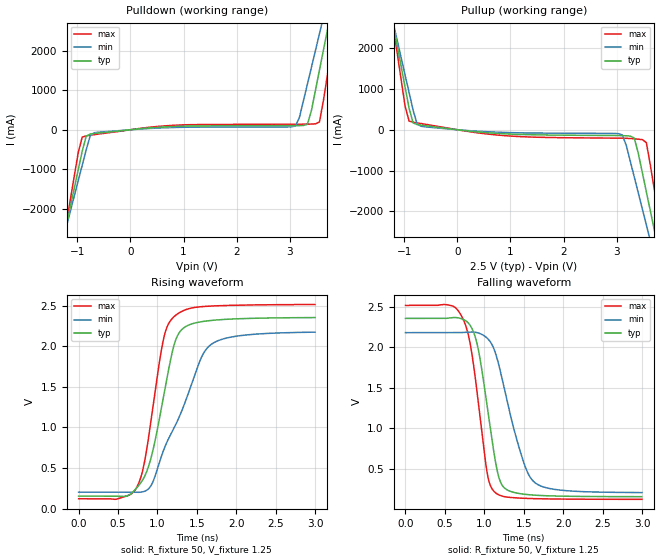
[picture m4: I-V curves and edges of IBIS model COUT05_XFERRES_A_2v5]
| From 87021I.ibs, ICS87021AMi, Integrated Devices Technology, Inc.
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[Model] COUT05_XFERRES_A_2v5
Model_type  Output
Polarity   Non-Inverting
Vmeas = 1.25
Rref = 50
Cref = 0
Vref = 1.25
|Variable  typ   min   max
C_comp   2p   1.5p   2.5p
[Voltage Range]   2.5   2.375   2.625
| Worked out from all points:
|   slope of the pulldown table from 0 to 0.375 V, typ, clamps not added: 7.84 ohm
|   slope of the pullup table from 0 to 0.375 V, typ, clamps not added: 7.17 ohm
|   rising waveform, R_fixture 50, V_fixture 1.25: 20-80 % time 274ps typ, 488ps min, 225ps max; typ from 0.154 V to 2.35 V
|   falling waveform, R_fixture 50, V_fixture 1.25: 20-80 % time 205ps typ, 309ps min, 191ps max; typ from 2.35 V to 0.154 V
| Open source, no load
|  Voltage   I(typ)   I(min)   I(max)
[Pullup]
-2.5V     11.44A     9.986A     13.84A
-1.212V   2.607A     2.64A      2.573A
-909.1mV  526mA      911.1mA    212mA
-833.3mV  167.1mA    478.9mA    184.4mA
-681.8mV  112.7mA    84.76mA    151.8mA
3.106V    -144.5mA   -124.8mA   -207.2mA
3.333V    -201.9mA   -1.16A     -222.3mA
3.485V    -1.051A    -1.943A    -242.2mA
3.561V    -1.521A    -2.334A    -315mA
3.712V    -2.464A    -3.118A    -1.472A
3.864V    -3.407A    -3.903A    -2.677A
5V        -10.49A    -9.798A    -11.71A
[Pulldown]
-2.5V     -10.49A    -9.183A    -12.66A
-1.288V   -2.917A    -2.872A    -3.01A
-1.212V   -2.443A    -2.477A    -2.405A
-909.1mV  -543.8mA   -898.7mA   -186.9mA
-833.3mV  -160.7mA   -504.4mA   -155.1mA
-757.6mV  -109mA     -149.4mA   -139.6mA
3.106V    103.9mA    93.06mA    139.6mA
3.333V    137.9mA    1.155A     141.5mA
3.561V    1.512A     2.434A     197.9mA
3.712V    2.539A     3.288A     1.405A
3.864V    3.567A     4.143A     2.72A
5V        11.31A     10.58A     12.63A
[Ramp]
|   typ   min   max
dV/dt_r   1.762/0.433n   1.577/0.660n   1.919/0.360n
dV/dt_f   1.769/0.311n   1.585/0.457n   1.923/0.297n
R_load =   50.0000
[Rising Waveform]
R_fixture = 50
V_fixture = 1.25   | VCC_typ
V_fixture_max = 1.3125   | VCC_max
V_fixture_min = 1.1875   | VCC_min
C_fixture = 0.0p
| Time   typ   min   max
0s        154.1mV    203.2mV    121.3mV
477.4ps   154.3mV    203.2mV    116.6mV
740.9ps   259.7mV    200.8mV    269.6mV
821.5ps   368.8mV    208.9mV    507.2mV
905.2ps   578.3mV    264.4mV    996.6mV
1.079ns   1.39V      722.9mV    2.098V
1.228ns   2.067V     1.027V     2.379V
1.553ns   2.301V     1.854V     2.487V
1.693ns   2.318V     2.03V      2.495V
2.998ns   2.352V     2.173V     2.513V
[Falling Waveform]
R_fixture = 50
V_fixture = 1.25   | VCC_typ
V_fixture_max = 1.3125   | VCC_max
V_fixture_min = 1.1875   | VCC_min
C_fixture = 0.0p
| Time   typ   min   max
0s        2.355V     2.179V     2.515V
725.4ps   2.344V     2.181V     2.356V
818.4ps   2.271V     2.187V     2.053V
911.4ps   2.026V     2.178V     1.415V
1.039ns   1.249V     2.109V     432mV
1.141ns   587mV      1.926V     202.8mV
1.259ns   258.4mV    1.464V     154.1mV
1.479ns   187.7mV    638mV      135.2mV
1.624ns   173.7mV    341.8mV    130.1mV
2.998ns   154.5mV    205mV      121.5mV
